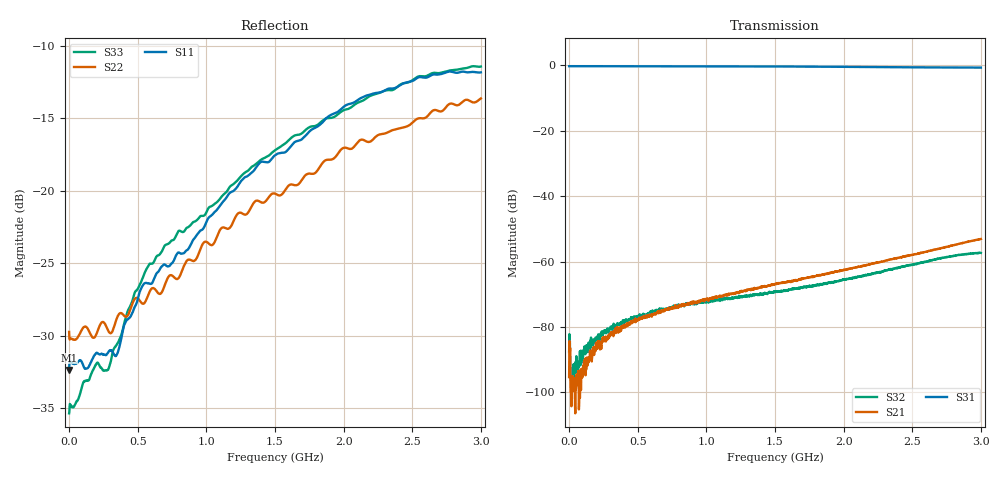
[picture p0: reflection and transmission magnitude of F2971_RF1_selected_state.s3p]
! Frequency:  300kHz to 3GHz
! Package:  4mm x 4mm LQFN Plastic Package: 20 pin with exposed paddle.
!  Pin 1,2,4,5,6,7,9,10,11,12,14,15,18,19 = GND
!  Pin 3  = RF1  = Port 1
!  Pin 8  = RFC  = Port 3
!  Pin 13 = RF2  = Port 2
!  Pin 16 = C2
!  Pin 17 = C1
!  Pin 20 = VDD
!  E.P.  = GND
! State:  RF1 Selected State
! Voltage:  VDD  = +3.0V
!  C1  = +3.0V (Logic HIGH)
!  C2  =  0V (Logic LOW)
! Data:  The device was measured on the F2971 EVKit using a calibrated
!  network analyzer. The results below remove the PCB trace and
!  connector effects using the Automatic Fixture Removal software
!  from Keysight. Therfore, the reference plane for these results
!  are at the device's RF pin.
! Misc:
! Date:  2018-03-27  SJ
! Note:
!  Integrated Device Technology supplies this data as a sample of
!  measured data. Data was taken at 25 degrees C. Integrated Device
!  Technology reserves the right to change this data at anytime.
# hz S db R 75
! 3 Port Network Data from SP1.SP block
! freq  dbS11  angS11  dbS12  angS12  dbS13  angS13
!  dbS21  angS21
!  dbS22  angS22  dbS23  angS23
!  dbS31  angS31  dbS32  angS32
!  dbS33  angS33
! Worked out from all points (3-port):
!   1601 points, 30 kHz to 3 GHz, reference 75 ohm
!   strongest paths, dB at 30 kHz, 750 MHz, 1.5 GHz, 2.25 GHz, 3 GHz:
!     S31: -0.2, -0.3, -0.3, -0.5, -0.7
!     S21: -95.3, -74.0, -67.0, -60.3, -53.1
!     S32: -87.7, -74.1, -69.2, -63.3, -57.3
!   lowest |S11| = -32.4 dB at 30 kHz (marker M1), VSWR 1.05, Z = 78.4 + j1.44 ohm
!   |S11| at or under -10 dB: start of sweep to end of sweep
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30000  -32.38 22.5  -82.05 100.4  -0.23 0.2
       -95.29 93.2  -29.75 174.5  -84.18 -54.1
       -0.23 0.2  -87.66 -58.1  -35.37 41.8
1.96903e8  -31.21 -34.5  -86.43 92.2  -0.23 -4.1
           -84.79 91.7  -29.95 -171.1  -83.93 70.6
           -0.23 -4.1  -83.60 68.0  -31.98 -39.9
2.831522e8  -31.19 -47.0  -83.53 99.2  -0.24 -5.8
            -82.99 92.7  -29.63 -160.7  -80.83 87.2
            -0.24 -5.8  -80.74 76.1  -32.37 -56.4
3.450266e8  -31.36 -60.5  -81.03 97.6  -0.24 -7.1
            -80.13 96.3  -28.88 -164.1  -79.81 81.0
            -0.24 -7.1  -80.27 83.7  -30.66 -67.7
3.806512e8  -30.19 -71.2  -80.23 100.4  -0.24 -7.8
            -79.94 100.3  -28.46 -158.4  -79.03 83.0
            -0.24 -7.8  -78.60 81.7  -29.94 -74.5
5.343997e8  -26.58 -83.7  -76.64 101.9  -0.25 -10.9
            -77.05 104.1  -27.80 -149.8  -76.54 83.3
            -0.25 -10.9  -76.20 84.6  -26.07 -84.7
6.99398e8  -25.11 -90.8  -74.53 104.1  -0.25 -14.3
           -74.52 102.6  -26.46 -148.9  -74.72 89.9
           -0.25 -14.3  -74.69 89.7  -23.77 -86.0
1.500015e9  -17.56 -116.7  -66.96 127.8  -0.30 -30.8
            -66.96 128.2  -20.21 -135.0  -69.10 117.8
            -0.31 -30.8  -69.18 115.9  -17.21 -106.1
2.154383e9  -13.48 -130.3  -61.18 141.3  -0.47 -44.3
            -61.16 141.8  -16.55 -134.1  -64.15 140.7
            -0.47 -44.3  -64.19 141.6  -13.71 -126.2
3e9  -11.84 -143.6  -53.06 143.6  -0.65 -60.8
     -53.07 143.5  -13.64 -135.1  -57.30 140.4
     -0.65 -60.8  -57.32 139.7  -11.44 -150.7
